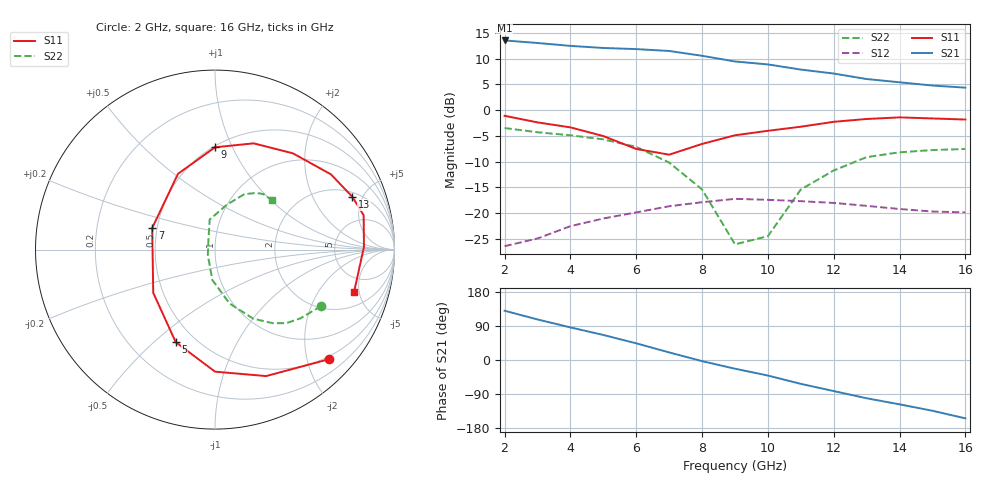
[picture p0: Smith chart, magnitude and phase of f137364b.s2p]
!ATF-13736
!S-PARAMETERS at Vds=4V  Id=40mA.  LAST UPDATED 07-22-92
# ghz s ma r 50
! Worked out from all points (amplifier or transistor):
!   15 points, 2 GHz to 16 GHz, reference 50 ohm
!   highest |S21| = 13.5 dB at 2 GHz (marker M1)
!   |S21| within 3 dB of that: start of sweep to 8.027 GHz
!   unconditionally stable (mu >= 1): 5.716 GHz to 9.066 GHz
!   at 4 GHz: K = 0.80, MSG = 17.5 dB, |S12| = -22.5 dB
!   at 9 GHz: K = 1.00, MAG = 13.2 dB, |S12| = -17.2 dB
!   at 16 GHz: K = 0.86, MSG = 12.1 dB, |S12| = -19.8 dB
!   S11 on the Smith chart (normalised r, x): 2 GHz: 0.44, -2.40; 5 GHz: 0.39, -0.59; 7 GHz: 0.47, +0.13; 9 GHz: 0.51, +0.86; 13 GHz: 2.32, +4.16; 16 GHz: 3.22, -4.43
2  0.88 -44.0  4.73 130.0  0.048 64.0  0.67 -28.0
3  0.76 -68.0  4.47 107.0  0.057 52.0  0.61 -39.0
4  0.68 -90.0  4.19 86.0  0.075 39.0  0.57 -46.0
5  0.56 -113.0  4 66.0  0.089 32.0  0.52 -52.0
6  0.42 -145.0  3.9 44.0  0.102 21.0  0.44 -61.0
7  0.37 161.0  3.74 20.0  0.117 9.0  0.31 -75.0
8  0.47 116.0  3.36 -3.0  0.128 -5.0  0.17 -95.0
9  0.57 90.0  2.96 -23.0  0.138 -19.0  0.05 -143.0
10  0.63 70.0  2.77 -41.0  0.135 -28.0  0.06 128.0
11  0.69 51.0  2.47 -63.0  0.131 -39.0  0.17 100.0
12  0.77 33.0  2.26 -82.0  0.126 -52.0  0.26 75.0
13  0.82 21.0  2 -101.0  0.118 -65.0  0.35 62.0
14  0.85 13.0  1.86 -117.0  0.11 -75.0  0.39 54.0
15  0.83 1.0  1.73 -134.0  0.104 -83.0  0.41 49.0
16  0.81 -17.0  1.65 -154.0  0.102 -103.0  0.42 41.0
